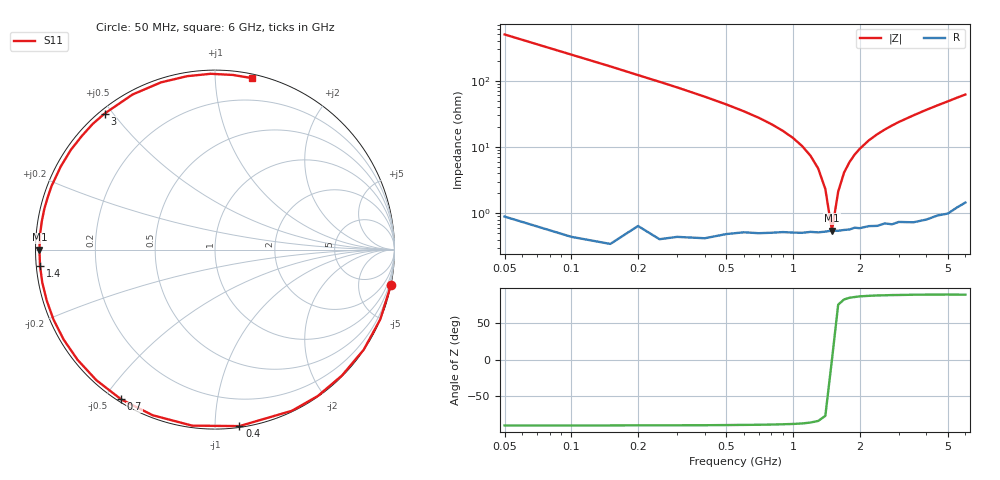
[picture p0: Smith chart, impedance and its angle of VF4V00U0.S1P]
! Infineon Technologies  Discrete & RF Semiconductors
! BBY 58-03
! Si Tuning Diode in SOD323
! VR = 4 V
! S-Parameters:  June  1999
# GHz  S  MA  R  50
!  f  S11
! GHz  MAG  ANG
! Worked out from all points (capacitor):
!   34 points, 50 MHz to 6 GHz, reference 50 ohm
!   read as one part to ground: C = 6.4 pF near 50 MHz
!   lowest |Z| = 552 mohm at 1.5 GHz (marker M1)
!   series resonance near 1.5 GHz, so ESL is about 1.8 nH
!   S11 on the Smith chart (normalised r, x): 50 MHz: 0.02, -9.93; 400 MHz: 0.01, -1.15; 700 MHz: 0.01, -0.55; 1.4 GHz: 0.01, -0.05; 3 GHz: 0.01, +0.48; 6 GHz: 0.03, +1.24
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0.05  0.9996 -11.5
0.1  0.9993 -22.9
0.15  0.9988 -33.9
0.2  0.9962 -44.8
0.25  0.9965 -54.9
0.3  0.995 -64.5
0.4  0.9927 -82.1
0.5  0.989 -97.4
0.6  0.986 -110.6
0.7  0.9847 -122.1
0.8  0.983 -132.3
0.9  0.9815 -141.3
1.1  0.9806 -156.6
1.2  0.9796 -163.2
1.4  0.979 -174.8
1.5  0.9781 -180.0
1.6  0.9784 175.3
1.8  0.9777 166.5
2  0.9771 158.8
2.4  0.9766 145.4
2.8  0.977 134.2
3  0.976 129.1
3.5  0.9786 118.0
4  0.9791 107.9
4.5  0.9786 99.1
5  0.9798 91.4
5.5  0.9782 84.1
6  0.9772 77.9
